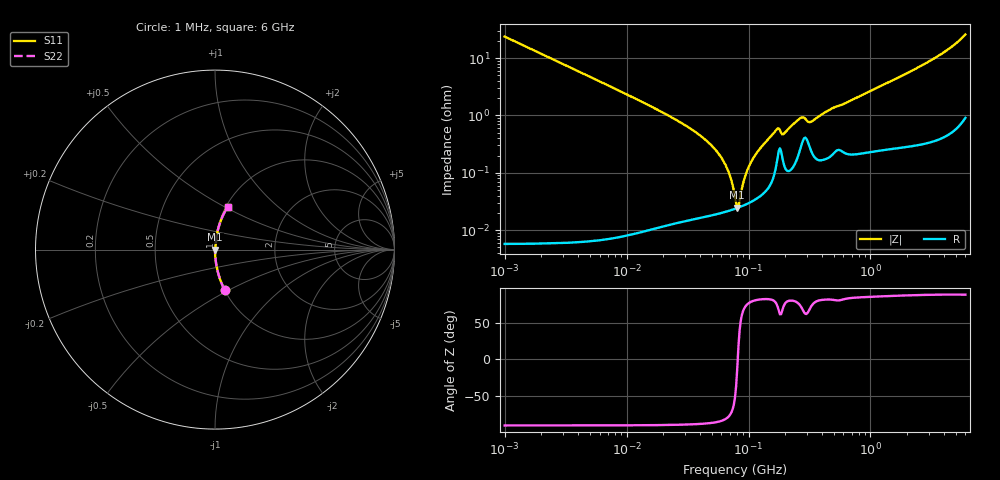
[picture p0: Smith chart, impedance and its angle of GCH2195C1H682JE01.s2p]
!Murata Part Number: GCH2195C1H682JE01
!These Parameters are Measured in Series Mode Connection
!Data Generated on Jun 19, 2026
!  o--ll--o
!Port1  Port2
!  o------o
!Operation Temp=25[degC], DC Bias Voltage=0[V]
!Freq. Start=1000[kHz] Stop=6[GHz] 401[Steps]
# Hz S RI R 50
!Freq.(Hz) S11(Real) S11(Imag) S21(Real) S21(Imag) S12(Real) S12(Imag) S22(Real) S22(Imag)
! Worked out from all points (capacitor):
!   401 points, 1 MHz to 6 GHz, reference 50 ohm
!   read as one part in series: C = 6.7 nF near 1.044 MHz
!   lowest |Z| = 24.8 mohm at 80.9 MHz (marker M1)
!   series resonance near 81.56 MHz, so ESL is about 570 pH
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1000000  0.0535 -0.225  0.9465 0.225  0.9465 0.225  0.0535 -0.225
4293785  0.0031 -0.055  0.9969 0.055  0.9969 0.055  0.0031 -0.055
1.843659e7  0.00026 -0.0122  0.9997 0.0122  0.9997 0.0122  0.00026 -0.0122
3.540316e7  0.000184 -0.00542  0.9998 0.00542  0.9998 0.00542  0.000184 -0.00542
5.236714e7  0.000193 -0.00266  0.9998 0.00266  0.9998 0.00266  0.000193 -0.00266
6.652088e7  0.000214 -0.0012  0.9998 0.0012  0.9998 0.0012  0.000214 -0.0012
7.256705e7  0.000226 -0.000684  0.9998 0.000684  0.9998 0.000684  0.000226 -0.000684
7.745967e7  0.000236 -0.000302  0.9998 0.000302  0.9998 0.000302  0.000236 -0.000302
8.090333e7  0.000244 -4.71e-05  0.9998 4.71e-05  0.9998 4.71e-05  0.000244 -4.71e-05
8.450008e7  0.000253 0.000208  0.9997 -0.000208  0.9997 -0.000208  0.000253 0.000208
9.420718e7  0.000279 0.000853  0.9997 -0.000853  0.9997 -0.000853  0.000279 0.000853
1.050294e8  0.000314 0.00152  0.9997 -0.00152  0.9997 -0.00152  0.000314 0.00152
1.223006e8  0.000386 0.00251  0.9996 -0.00251  0.9996 -0.00251  0.000386 0.00251
1.658303e8  0.00114 0.00521  0.9989 -0.00521  0.9989 -0.00521  0.00114 0.00521
1.732027e8  0.00188 0.00559  0.9981 -0.00559  0.9981 -0.00559  0.00188 0.00559
1.973453e8  0.00131 0.00475  0.9987 -0.00475  0.9987 -0.00475  0.00131 0.00475
2.734687e8  0.00326 0.00861  0.9967 -0.00861  0.9967 -0.00861  0.00326 0.00861
3.325952e8  0.00224 0.00762  0.9978 -0.00762  0.9978 -0.00762  0.00224 0.00762
4.813793e8  0.00218 0.013  0.9978 -0.013  0.9978 -0.013  0.00218 0.013
1.428092e9  0.00402 0.0381  0.996 -0.0381  0.996 -0.0381  0.00402 0.0381
3.483508e9  0.0144 0.1027  0.9856 -0.1027  0.9856 -0.1027  0.0144 0.1027
6e9  0.0698 0.2378  0.9302 -0.2378  0.9302 -0.2378  0.0698 0.2378
